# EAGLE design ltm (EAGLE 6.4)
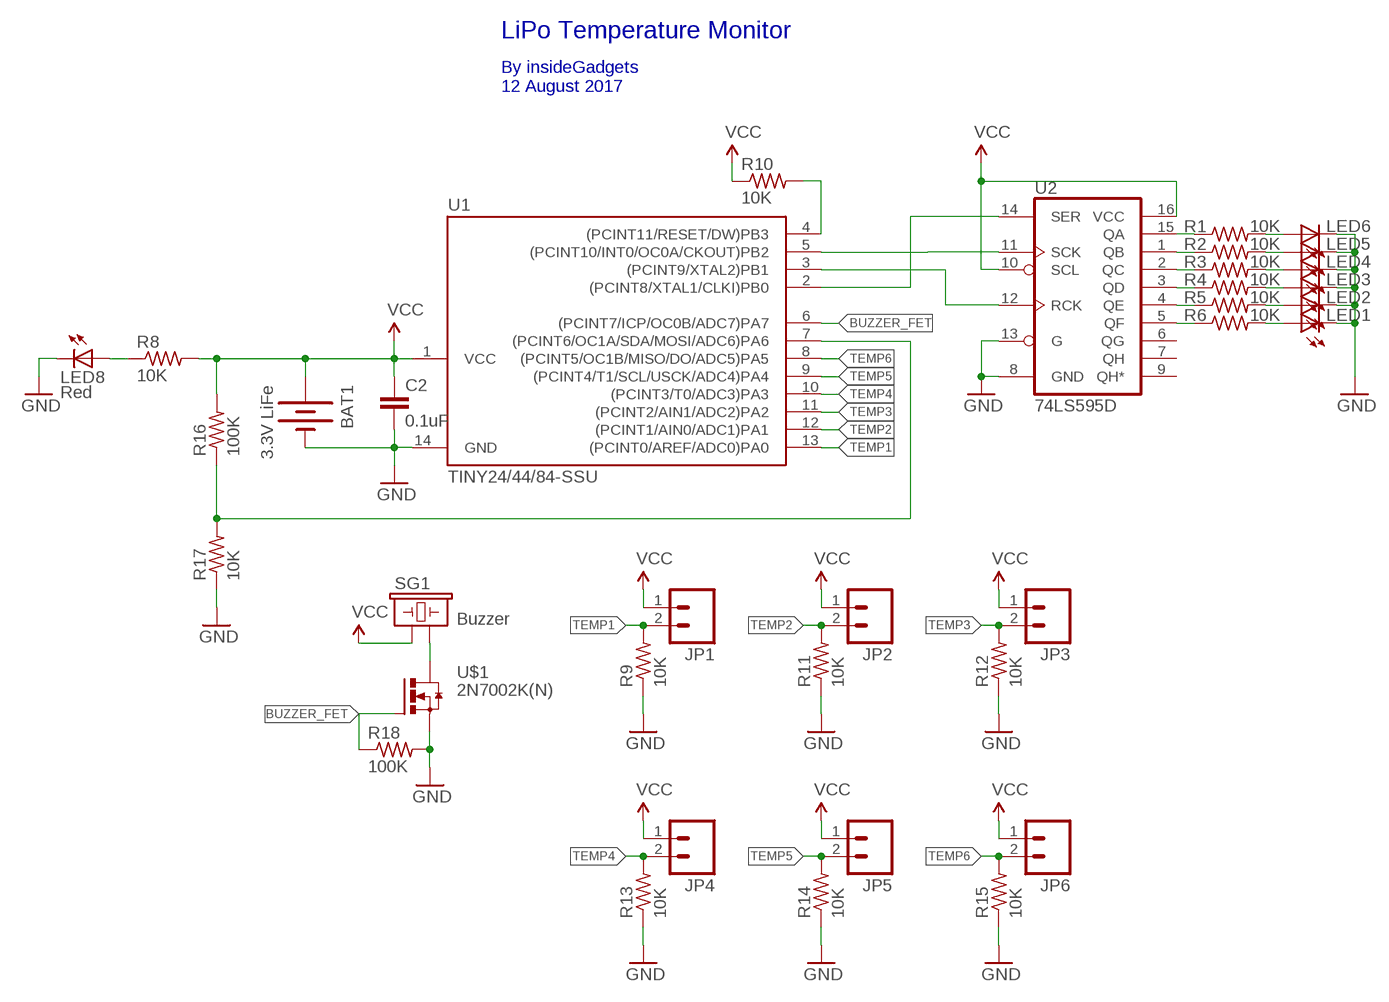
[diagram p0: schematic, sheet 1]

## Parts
BAT1  3.3V LiFe  BATTERYAA-RS  [BATTERY-AA-RS]
C2  0.1uF  CAP0805  [C0805K]
JP1  M021X2-EBAY  [MOLEX-1X2-EBAY]
JP2  M021X2-EBAY  [MOLEX-1X2-EBAY]
JP3  M021X2-EBAY  [MOLEX-1X2-EBAY]
JP4  M021X2-EBAY  [MOLEX-1X2-EBAY]
JP5  M021X2-EBAY  [MOLEX-1X2-EBAY]
JP6  M021X2-EBAY  [MOLEX-1X2-EBAY]
LED1  Red  LEDCHIP-LED0805  [CHIP-LED0805]
LED2  Red  LEDCHIP-LED0805  [CHIP-LED0805]
LED3  Red  LEDCHIP-LED0805  [CHIP-LED0805]
LED4  Red  LEDCHIP-LED0805  [CHIP-LED0805]
LED5  Red  LEDCHIP-LED0805  [CHIP-LED0805]
LED6  Red  LEDCHIP-LED0805  [CHIP-LED0805]
LED8  Red  LEDCHIP-LED0805  [CHIP-LED0805]
R1  10K  R-US_R0805_2  [R0805_2]
R2  10K  R-US_R0805_2  [R0805_2]
R3  10K  R-US_R0805_2  [R0805_2]
R4  10K  R-US_R0805_2  [R0805_2]
R5  10K  R-US_R0805_2  [R0805_2]
R6  10K  R-US_R0805_2  [R0805_2]
R8  10K  R-US_R0805_2  [R0805_2]
R9  10K  R-US_R0805_2  [R0805_2]
R10  10K  R-US_R0805_2  [R0805_2]
R11  10K  R-US_R0805_2  [R0805_2]
R12  10K  R-US_R0805_2  [R0805_2]
R13  10K  R-US_R0805_2  [R0805_2]
R14  10K  R-US_R0805_2  [R0805_2]
R15  10K  R-US_R0805_2  [R0805_2]
R16  100K  R-US_R0805_2  [R0805_2]
R17  10K  R-US_R0805_2  [R0805_2]
R18  100K  R-US_R0805_2  [R0805_2]
SG1  Buzzer  BUZZER7MMPITCH  [BUZZER-12MM-7MMPITCH]
U1  TINY24/44/84-SSU  [SOIC14]
U2  74LS595D  [SO16]
U$1  2N7002K(N)  2N7002K_(N)SOT-23  [SOT-23]

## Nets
BUZZER_FET: R18.1 U1.6((PCINT7/ICP/OC0B/ADC7)PA7) U$1.1(G)
GND: BAT1.GND@2(-) C2.2 LED1.C LED2.C LED3.C LED4.C LED5.C LED6.C LED8.C R9.1 R11.1 R12.1 R13.1 R14.1 R15.1 R17.1 R18.2 U1.14(GND) U2.8(GND) U2.13(G) U$1.2(S)
N$1: LED6.A R1.2
N$2: R1.1 U2.15(QA)
N$3: LED5.A R2.2
N$4: LED8.A R8.1
N$5: LED4.A R3.2
N$6: U1.3((PCINT9/XTAL2)PB1) U2.12(RCK)
N$7: LED3.A R4.2
N$8: R6.1 U2.5(QF)
N$9: LED2.A R5.2
N$10: R5.1 U2.4(QE)
N$11: LED1.A R6.2
N$12: R4.1 U2.3(QD)
N$13: U1.5((PCINT10/INT0/OC0A/CKOUT)PB2) U2.11(SCK)
N$14: R3.1 U2.2(QC)
N$15: U1.2((PCINT8/XTAL1/CLKI)PB0) U2.14(SER)
N$16: R2.1 U2.1(QB)
N$17: R16.1 R17.2 U1.7((PCINT6/OC1A/SDA/MOSI/ADC6)PA6)
N$18: SG1.- U$1.3(D)
RESET: R10.2 U1.4((PCINT11/RESET/DW)PB3)
TEMP1: JP1.2 R9.2 U1.13((PCINT0/AREF/ADC0)PA0)
TEMP2: JP2.2 R11.2 U1.12((PCINT1/AIN0/ADC1)PA1)
TEMP3: JP3.2 R12.2 U1.11((PCINT2/AIN1/ADC2)PA2)
TEMP4: JP4.2 R13.2 U1.10((PCINT3/T0/ADC3)PA3)
TEMP5: JP5.2 R14.2 U1.9((PCINT4/T1/SCL/USCK/ADC4)PA4)
TEMP6: JP6.2 R15.2 U1.8((PCINT5/OC1B/MISO/DO/ADC5)PA5)
VCC: BAT1.PWR@2(+) C2.1 JP1.1 JP2.1 JP3.1 JP4.1 JP5.1 JP6.1 R8.2 R10.1 R16.2 SG1.+ U1.1(VCC) U2.10(SCL) U2.16(VCC)
Unconnected: U2.6(QG) U2.7(QH) U2.9(QH*)

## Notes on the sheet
- LiPo Temperature Monitor
- By insideGadgets
  12 August 2017

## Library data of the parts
BAT1 = SparkFun:BATTERY: Battery Holders
C2 = adafruit:CAP
JP1-JP6 = SparkFun:M02: Header 2
LED1-LED6 LED8 = adafruit:LED: LED
R1-R6 R8-R18 = adafruit:R-US_: RESISTOR, American symbol
SG1 = SparkFun:BUZZER: Buzzer 12mm
U1 = avr-5:TINY24/44/84
U2 = SparkFun:74*595: 8-bit SHIFT REGISTER, output latch
U$1 = alex:2N7002K_(N)

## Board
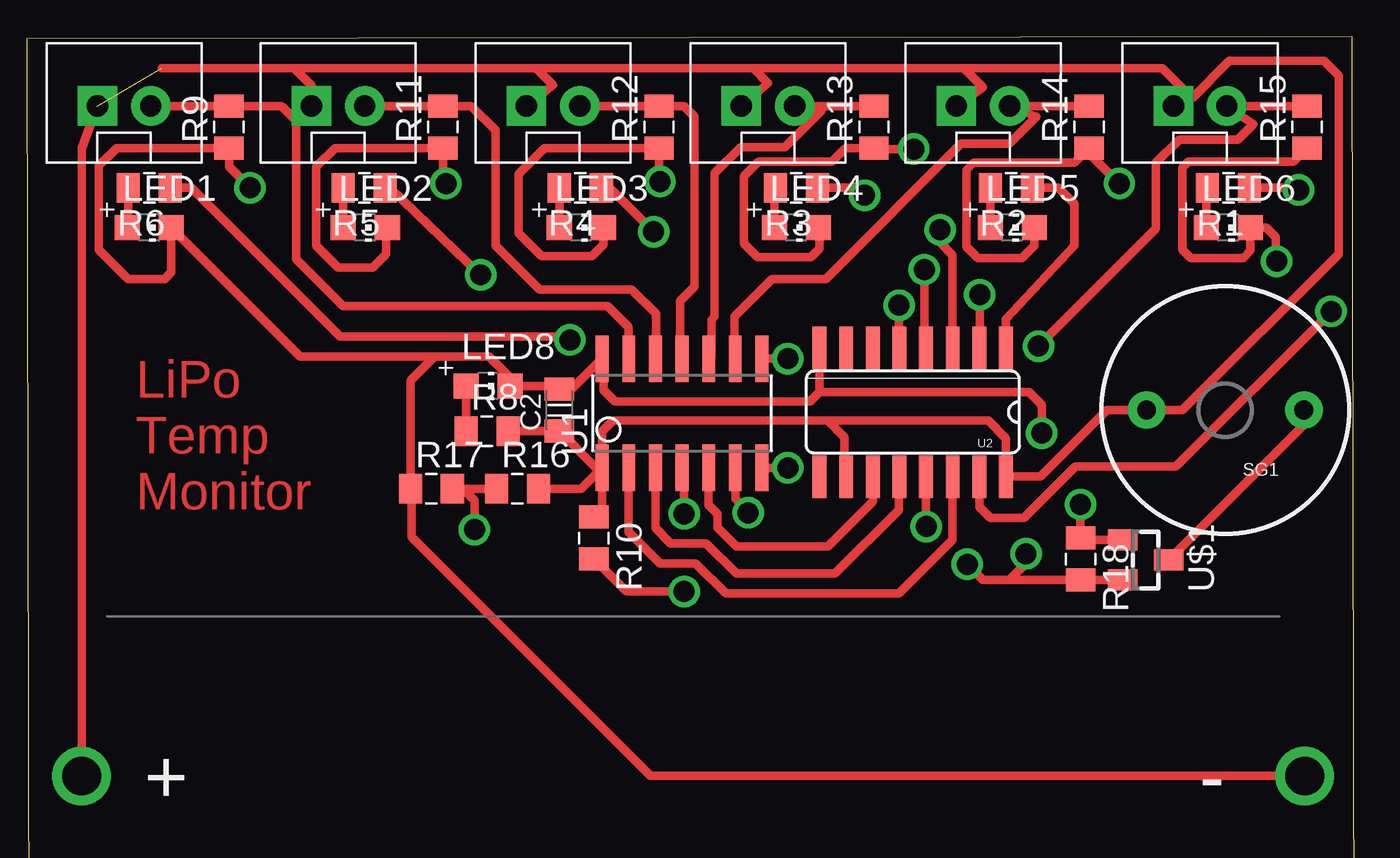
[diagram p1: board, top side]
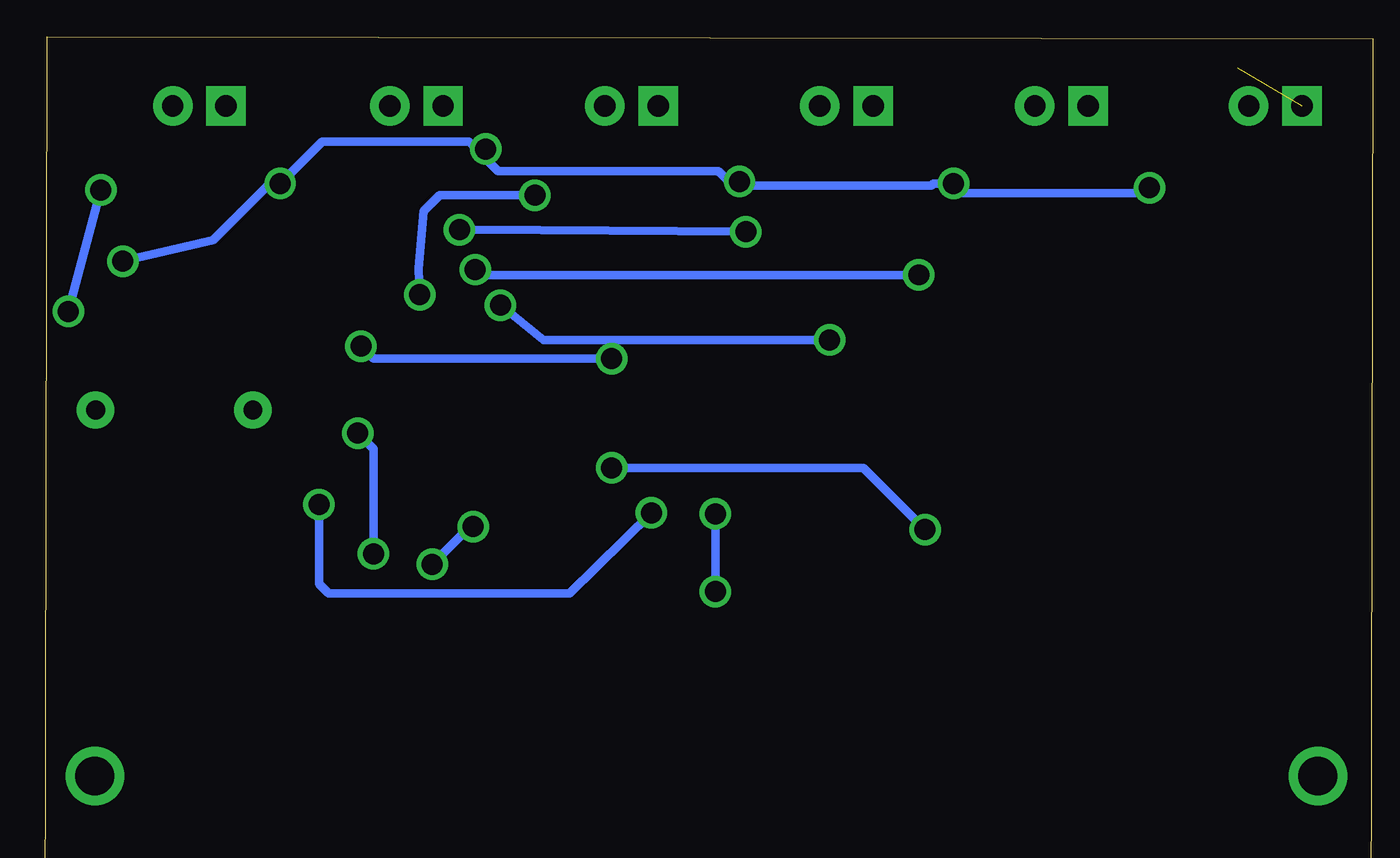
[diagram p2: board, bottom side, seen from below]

No outline drawn. Coordinates in mm, seen from the top.
Copper layers (1*16): Top 0.035mm / dielectric 1.5mm / Bottom 0.035mm
Design rules "Fusion_eagle_rule_v1.1": minimum track width 6mil, minimum drill 12mil, track to track 6mil, track to pad 6mil, pad to pad 6mil, via to via 6mil, smd to smd 0mil, copper to edge 10mil, drill to drill 10mil, minimum pad ring 10mil, minimum via ring 6mil, stop-mask expansion 2mil, vias tented up to drill 100mil, thermal gap 10mil
Milling: 4 lines

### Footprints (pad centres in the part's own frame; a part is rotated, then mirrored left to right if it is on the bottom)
BATTERY-AA-RS = drill 1.854: GND@2 40.586,0; PWR@2 -17.726,0
C0805K = smd 1.1 x 1.4: 1 -1,0; 2 1,0
MOLEX-1X2-EBAY = drill 1.016 pad 1.88 square: 1 -1.27,0 | drill 1.016 pad 1.88: 2 1.27,0
CHIP-LED0805 = smd 1.2 x 1.2: A 0,-1.05; C 0,1.05
R0805_2 = smd 1.1 x 1.4: 1 -1,0; 2 1,0
BUZZER-12MM-7MMPITCH = drill 0.9 pad 1.778: + 3.75,0; - -3.75,0
SOIC14 = smd 0.61 x 2.21: 1 -3.81,-2.603; 2 -2.54,-2.603; 3 -1.27,-2.603; 4 0,-2.603; 5 1.27,-2.603; 6 2.54,-2.603; 7 3.81,-2.603; 8 3.81,2.603; 9 2.54,2.603; 10 1.27,2.603; 11 0,2.603; 12 -1.27,2.603; 13 -2.54,2.603; 14 -3.81,2.603
SO16 = smd 0.66 x 2.032: 1 -4.445,-3.073; 2 -3.175,-3.073; 3 -1.905,-3.073; 4 -0.635,-3.073; 5 0.635,-3.073; 6 1.905,-3.073; 7 3.175,-3.073; 8 4.445,-3.073; 9 4.445,3.073; 10 3.175,3.073; 11 1.905,3.073; 12 0.635,3.073; 13 -0.635,3.073; 14 -1.905,3.073; 15 -3.175,3.073; 16 -4.445,3.073
SOT-23 = smd 1 x 1.4: 1 -0.95,-1.1; 2 0.95,-1.1; 3 0,1.1

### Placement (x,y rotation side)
BAT1  20.25,8.65 0 top
C2  25.3,26.1 90 top
JP1  4.55,40.6 0 top
JP2  14.75,40.6 0 top
JP3  25,40.6 0 top
JP4  35.25,40.6 0 top
JP5  45.5,40.6 0 top
JP6  55.85,40.6 0 top
LED1  5.75,34.8 270 top
LED2  16.05,34.8 270 top
LED3  26.35,34.8 270 top
LED4  36.6,34.8 270 top
LED5  46.9,34.8 270 top
LED6  57.2,34.8 270 top
LED8  21.9,27.25 270 top
R1  57.2,36.7 180 top
R2  46.85,36.7 180 top
R3  36.6,36.7 180 top
R4  26.3,36.7 180 top
R5  16,36.7 180 top
R6  5.75,36.7 180 top
R8  21.85,25.1 0 top
R9  9.55,39.6 90 top
R10  26.95,20 270 top
R11  19.75,39.6 90 top
R12  30.05,39.6 90 top
R13  40.3,39.6 90 top
R14  50.55,39.6 90 top
R15  60.95,39.6 90 top
R16  23.3,22.35 0 top
R17  19.2,22.35 0 top
R18  50.15,19 270 top
SG1  57.05,26.1 180 top
U1  31.15,25.95 0 top
U2  42.15,26 180 top
U$1  53.25,18.95 270 top

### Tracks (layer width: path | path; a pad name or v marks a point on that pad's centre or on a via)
BUZZER_FET  (via drill 1)
  Top 0.406: U$1.1 50.25,19.9 R18.1 v50.15,21.6 | U1.6 33.69,21.86 v34.3,21.2
  Bottom 0.406: v34.3,21.2 38.2,17.35 49.7,17.35 50.15,17.8 v50.15,21.6
GND  (via drill 1)
  Top 0.406: 42.75,22.71 U2.13 42.78,20.91 v42.8,20.55 | 19.35,28.65 12.95,28.65 LED1.C 6.8,32.7 6.45,32.35 | 19.35,28.65 21.95,28.65 22.95,27.65 LED8.C 25.15,27.25 C2.2 25.89,27.1 U1.14 27.4,28.49 27.4,27.05 27.95,26.5 37.25,26.5 37.7,26.95 | U2.8 37.7,26.95 | 19.35,28.65 18.2,27.5 R17.1 18.25,22.3 18.25,20.05 29.65,8.65 BAT1.GND@2 | 37.7,26.95 47.7,26.95 48.3,26.35 v48.3,25 | R18.2 U$1.2 46.75,18 | 46.75,18 45.5,18 v44.75,18.75 | v47.55,19.25 47.55,18.8 46.75,18 | 27.4,34.7 LED3.C 27.4,34 26.85,33.45 24.45,33.45 23.35,34.55 23.35,37.35 24.6,38.6 R12.1 30.05,37.05 v30.1,37 | 6.45,32.35 4.75,32.35 3.35,33.75 3.35,37.75 4.2,38.6 R9.1 9.55,38.1 | 6.45,32.35 6.5,32.35 6.8,32.65 | LED4.C 37.7,34.75 37.7,33.8 37.3,33.4 34.75,33.4 34.1,34.05 34.1,37.25 34.8,37.95 38.3,37.95 38.95,38.6 R13.1 40.35,38.55 v42.2,38.55 | 9.55,38.1 9.55,37.7 v10.55,36.7 | v19.9,36.9 19.75,37.05 R11.1 14.6,38.6 13.7,37.7 13.7,33.95 14.75,32.9 16.4,32.9 17.05,33.55 17.05,34.75 LED2.C | LED5.C 47.95,33.95 47.35,33.35 45.25,33.35 44.7,33.9 44.7,37.55 45.05,37.9 49.85,37.9 R14.1 50.55,38.35 v52,36.9 | R15.1 60.3,37.95 55.3,37.95 55,37.65 55,33.75 55.4,33.35 57.9,33.35 58.25,33.7 LED6.C 59,34.8 59.45,34.35 59.45,33.25 v59.5,33.2 | 9.6,38.6 9.6,38.15 9.55,38.1
  Bottom 0.406: v42.8,20.55 42.8,20.7 v44.75,18.75 | v48.3,25 47.55,24.25 v47.55,19.25 | v10.55,36.7 10.65,37.05 11.25,36.45 19.95,36.45 20.4,36.9 | v19.9,36.9 20.4,36.9 | 20.4,36.9 20.85,36.9 20.95,36.8 29.9,36.8 v30.1,37 30.6,37 31.1,37.5 41.6,37.5 42.65,38.55 | v42.2,38.55 42.65,38.55 | 42.65,38.55 43,38.9 50,38.9 v52,36.9 52.5,36.9 55.2,34.2 v59.5,33.2
N$1
  Top 0.406: R1.2 56.15,36.65 LED6.A
N$2  (via drill 1)
  Top 0.406: 45.45,22.8 U2.15 45.33,21.48 45.85,20.95 47.45,20.95 49.9,23.4 54.7,23.4 v62.1,30.8 | R1.1 60.45,36.7 v60.55,36.6
  Bottom 0.406: v62.1,30.8 v60.55,36.6
N$3
  Top 0.406: R2.2 LED5.A
N$4
  Top 0.406: LED8.A R8.1
N$5
  Top 0.406: R3.2 35.55,36.65 LED4.A
N$6
  Top 0.406: U1.3 29.88,20.47 30.6,19.75 32.3,19.75 33.75,18.3 38.45,18.3 41.5,21.35 41.5,22.91 U2.12
N$7
  Top 0.406: R4.2 LED3.A
N$8  (via drill 1)
  Top 0.406: R6.1 7.75,36.7 14.85,29.6 25.65,29.6 v25.8,29.45 | v41.5,31.1 41.5,28.4 41.65,28.25 41.65,28.69 U2.5
  Bottom 0.406: v25.8,29.45 39.45,29.45 v41.5,31.1
N$9
  Top 0.406: R5.2 LED2.A
N$10  (via drill 1)
  Top 0.406: R5.1 17.2,36.7 v21.55,32.55 | v42.7,32.8 42.7,28.91 U2.4
  Bottom 0.406: v21.55,32.55 42.65,32.55 v42.7,32.8
N$11
  Top 0.406: R6.2 4.75,34.85 LED1.A
N$12  (via drill 1)
  Top 0.406: U2.3 44.05,28.83 44.05,33.5 43.45,34.1 v43.45,34.7 | R4.1 27.7,36.7 v29.8,34.6
  Bottom 0.406: v29.8,34.6 42.85,34.7 v43.45,34.7
N$13
  Top 0.406: 40.25,22.67 U2.11 40.25,21.75 38.1,19.6 33.75,19.6 32.85,20.5 32.85,21.15 32.42,21.58 U1.5
N$14  (via drill 1)
  Top 0.406: R3.1 39.35,36.7 39.4,36.75 39.45,36.75 v39.85,36.35 | v45.35,31.6 45.35,28.85 U2.2
  Bottom 0.406: v39.85,36.35 44.4,36.35 45.15,35.6 45.4,32.85 v45.35,31.6
N$15
  Top 0.406: U1.2 28.61,20.29 30.1,18.8 31.8,18.8 33.25,17.35 41.5,17.35 44.05,19.9 U2.14
N$16
  Top 0.406: R2.1 49.1,36.7 49.85,35.95 49.85,33.95 46.6,30.45 46.6,28.83 U2.1
N$17  (via drill 1)
  Top 0.406: R17.2 20.7,22.35 | 20.7,22.35 R16.1 | U1.7 v36.2,23.35 | v21.25,20.4 21.25,21.8 20.7,22.35
  Bottom 0.406: v36.2,23.35 24.2,23.35 v21.25,20.4
N$18
  Top 0.406: U$1.3 60.8,25.4 SG1.-
RESET  (via drill 1)
  Top 0.406: v31.25,21.15 31.25,23.25 U1.4 | R10.2 28.5,17.45 v31.25,17.45
  Bottom 0.406: v31.25,17.45 v31.25,21.15
TEMP1
  Top 0.406: JP1.2 R9.2 12.05,40.6 12.75,39.9 12.75,33.3 15,31.05 27.6,31.05 28.6,30.05 28.6,28.56 U1.13
TEMP2
  Top 0.406: JP2.2 R11.2 21.1,40.6 22.25,39.45 22.25,33.95 24.35,31.85 28.75,31.85 29.9,30.7 29.9,28.57 U1.12
TEMP3
  Top 0.406: JP3.2 R12.2 31.25,40.6 31.75,40.1 31.75,32 31.05,31.3 31.05,28.65 U1.11
TEMP4
  Top 0.406: R13.2 JP4.2 37.79,40.39 36.05,38.65 33.95,38.65 32.7,37.4 32.7,30.55 32.55,30.4 32.55,28.68 U1.10
TEMP5
  Top 0.406: R14.2 JP5.2 48.04,40.09 46.75,38.8 44.45,38.8 38,32.35 35.45,32.35 33.65,30.55 33.65,28.59 U1.9
TEMP6  (via drill 1)
  Top 0.406: R15.2 JP6.2 58.39,39.74 57.65,39 54.85,39 53.75,37.9 53.75,34.75 v48.15,29.15 | U1.8 36.1,28.55 v36.2,28.55
  Bottom 0.406: v36.2,28.55 47.55,28.55 v48.15,29.15
VCC  (1 unrouted)
  Top 0.406: 6.35,42.4 12.65,42.4 | 12.65,42.4 24.2,42.4 | 24.2,42.4 34.55,42.4 | 34.55,42.4 44.6,42.4 | 44.6,42.4 54.05,42.4 55.48,40.98 | 55.48,40.98 JP6.1 | JP4.1 35.25,41.7 34.55,42.4 | JP3.1 25,41.6 24.2,42.4 | JP5.1 45.5,41.5 44.6,42.4 | U1.1 27.05,23.35 C2.1 R8.2 | JP1.1 2.52,38.57 BAT1.PWR@2 | 38.85,22.8 U2.10 38.9,22.75 38.9,24.8 38.1,25.6 | U1.1 27.34,25.09 27.85,25.6 38.1,25.6 | 38.1,25.6 45.75,25.6 46.59,24.75 U2.16 48.23,22.93 51.4,26.1 SG1.+ 55,26.1 62.45,33.55 62.45,42.05 61.75,42.75 57.25,42.75 55.48,40.98 | R16.2 26.34,22.35 U1.1 | R10.1 27.34,21.39 U1.1 | JP2.1 13.48,41.57 12.65,42.4

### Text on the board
Top: LiPo / Temp / Monitor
